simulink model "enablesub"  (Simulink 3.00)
settings: Solver=VariableStepDiscrete  StartTime=0.0  StopTime=10.0  RelTol=1e-3
libraries: simulink3 x1

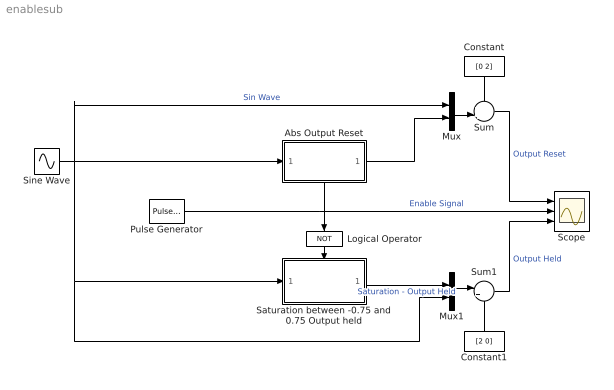
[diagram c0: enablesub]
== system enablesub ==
  Abs Output Reset : Subsystem
  Constant : Constant  Orientation=down  Value=[0 2]
  Constant1 : Constant  Orientation=up  Value=[2 0]
  Logical Operator : Logic  Orientation=down  Operator=NOT  Inputs=1
  Mux : Mux  Inputs=2
  Mux1 : Mux  Inputs=2
  Pulse Generator : simulink3/Sources/Pulse Generator  period=5  duty=50  amplitude=1  start=0
  Saturation between -0.75 and 0.75 Output held : Subsystem
  Scope : Scope  NumInputPorts=3
  Sine Wave : Sin  Amplitude=1  Frequency=1  Phase=0  SampleTime=0
  Sum : Sum  Inputs=++|  SaturateOnIntegerOverflow=on
  Sum1 : Sum  Inputs=|++  SaturateOnIntegerOverflow=on
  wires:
  Sine Wave/1 -> Abs Output Reset/1(In), Mux/1, Saturation between -0.75 and 0.75 Output held/1(In), Mux1/2  "Sin Wave"
  Saturation between -0.75 and 0.75 Output held/1(Out) -> Mux1/1  "Saturation - Output Held"
  Logical Operator/1 -> Saturation between -0.75 and 0.75 Output held/Enable
  Constant/1 -> Sum/1
  Mux/1 -> Sum/2
  Abs Output Reset/1(Out) -> Mux/2
  Sum/1 -> Scope/1  "Output Reset"
  Mux1/1 -> Sum1/1
  Constant1/1 -> Sum1/2
  Pulse Generator/1 -> Logical Operator/1, Scope/2, Abs Output Reset/Enable  "Enable Signal"
  Sum1/1 -> Scope/3  "Output Held"

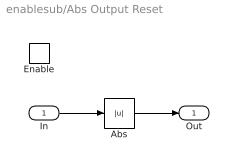
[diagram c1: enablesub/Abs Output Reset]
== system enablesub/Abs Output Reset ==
  In : Inport  Port=1  PortWidth=-1  SampleTime=-1  DataType=auto
  Enable : EnablePort  StatesWhenEnabling=reset
  Abs : Abs
  Out : Outport  Port=1  OutputWhenDisabled=reset  InitialOutput=0
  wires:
  In/1 -> Abs/1
  Abs/1 -> Out/1

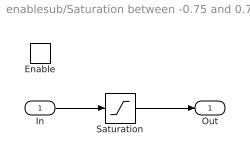
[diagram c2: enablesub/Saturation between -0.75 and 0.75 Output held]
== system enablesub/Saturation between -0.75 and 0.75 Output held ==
  In : Inport  Port=1  PortWidth=-1  SampleTime=-1  DataType=auto
  Enable : EnablePort
  Saturation : Saturate  UpperLimit=0.75  LowerLimit=-0.75
  Out : Outport  Port=1
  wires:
  Saturation/1 -> Out/1
  In/1 -> Saturation/1
